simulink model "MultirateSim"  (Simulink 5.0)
settings: Solver=ode45  StartTime=0.0  StopTime=2  RelTol=1e-3
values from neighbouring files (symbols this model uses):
  AL = A^L    [Multirate.m]
  BL = [A^i*B,BL]    [Multirate.m]
  CL = [CL;C*A^i]    [Multirate.m]
  DL = zeros(L,L)    [Multirate.m]
undefined symbols (not defined in the file or in its folder): denDc, numDc

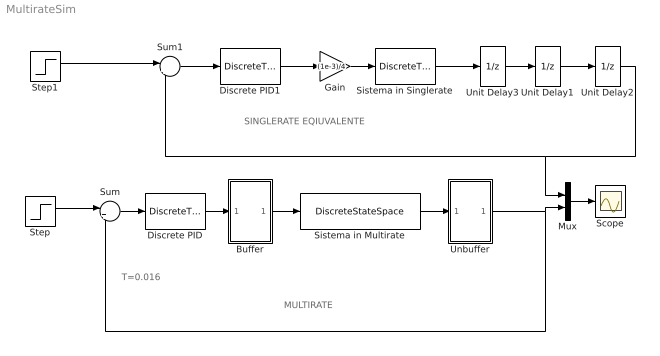
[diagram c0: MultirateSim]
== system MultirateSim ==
  note: MULTIRATE
  note: SINGLERATE EQIUVALENTE
  note: T=0.016
  Buffer : Subsystem
  Discrete PID : DiscreteTransferFcn  Numerator=numDc  Denominator=denDc  SampleTime=0.004
  Discrete PID1 : DiscreteTransferFcn  Numerator=numDc  Denominator=denDc  SampleTime=0.016
  Gain : Gain  Gain=(1e-3)/4
  Mux : Mux  Inputs=2
  Scope : Scope
  Sistema in Singlerate : DiscreteTransferFcn  Numerator=[211.04 63.62 0]  Denominator=[1 -1.776 0.7864]  SampleTime=0.016
  Sistema in Multirate : DiscreteStateSpace  A=AL  B=BL  C=CL  D=DL  SampleTime=0.016
  Step : Step  Time=0  SampleTime=0.016
  Step1 : Step  Time=0  SampleTime=0.016
  Sum : Sum  Inputs=|+-
  Sum1 : Sum  Inputs=|+-
  Unbuffer : Subsystem
  Unit Delay1 : UnitDelay  SampleTime=0.004
  Unit Delay2 : UnitDelay  SampleTime=0.004
  Unit Delay3 : UnitDelay  SampleTime=0.004
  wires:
  Step/1 -> Sum/1
  Sum/1 -> Discrete PID/1
  Discrete PID/1 -> Buffer/1(In1)
  Buffer/1(Out1) -> Sistema in Multirate/1
  Sistema in Multirate/1 -> Unbuffer/1(In1)
  Unbuffer/1(Out1) -> Sum/2, Mux/2
  Mux/1 -> Scope/1
  Sum1/1 -> Discrete PID1/1
  Discrete PID1/1 -> Gain/1
  Step1/1 -> Sum1/1
  Sistema in Singlerate/1 -> Unit Delay3/1
  Unit Delay3/1 -> Unit Delay1/1
  Gain/1 -> Sistema in Singlerate/1
  Unit Delay1/1 -> Unit Delay2/1
  Unit Delay2/1 -> Sum1/2, Mux/1

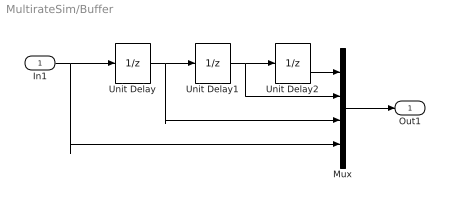
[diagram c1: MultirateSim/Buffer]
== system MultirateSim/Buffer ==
  In1 : Inport
  Mux : Mux
  Unit Delay : UnitDelay  SampleTime=0.004
  Unit Delay1 : UnitDelay  SampleTime=0.004
  Unit Delay2 : UnitDelay  SampleTime=0.004
  Out1 : Outport
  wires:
  Unit Delay/1 -> Unit Delay1/1, Mux/3
  Unit Delay1/1 -> Unit Delay2/1, Mux/2
  In1/1 -> Mux/4, Unit Delay/1
  Unit Delay2/1 -> Mux/1
  Mux/1 -> Out1/1

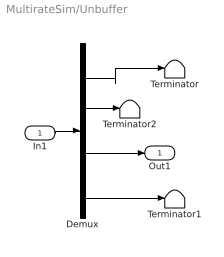
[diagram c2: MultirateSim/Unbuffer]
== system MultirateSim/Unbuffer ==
  In1 : Inport
  Demux : Demux
  Terminator : Terminator
  Terminator1 : Terminator
  Terminator2 : Terminator
  Out1 : Outport
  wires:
  Demux/2 -> Terminator2/1
  Demux/3 -> Out1/1
  In1/1 -> Demux/1
  Demux/4 -> Terminator1/1
  Demux/1 -> Terminator/1
